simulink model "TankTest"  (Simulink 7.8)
settings: Solver=ode45  StartTime=0.0  StopTime=SimulationPeriod  RelTol=1e-7
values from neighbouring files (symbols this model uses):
  Ar1 = 1*2    (= 2)    [runSim.m]
  Ar2 = 0.6666667*2    (= 1.3333334)    [runSim.m]
  BT = 250-10*abs(8-i)    [runSim.m]
  g = 9.8    [runSim.m]
  h_add = 0.2    [runSim.m]
  k1 = 4.88e-4    (= 0.000488)    [runSim.m]
  k2 = 3.177e-4    (= 0.0003177)    [runSim.m]
  levelR1 = 1    [runSim.m]
  levelR2 = 0.75    [runSim.m]
  openloop = false    [runSim.m]
  qh0 = 0.01    [runSim.m]
  rho = 800    [runSim.m]
  Ttarget = 200    [runSim.m]
  UA0 = 100    [runSim.m]
undefined symbols (not defined in the file or in its folder): cp

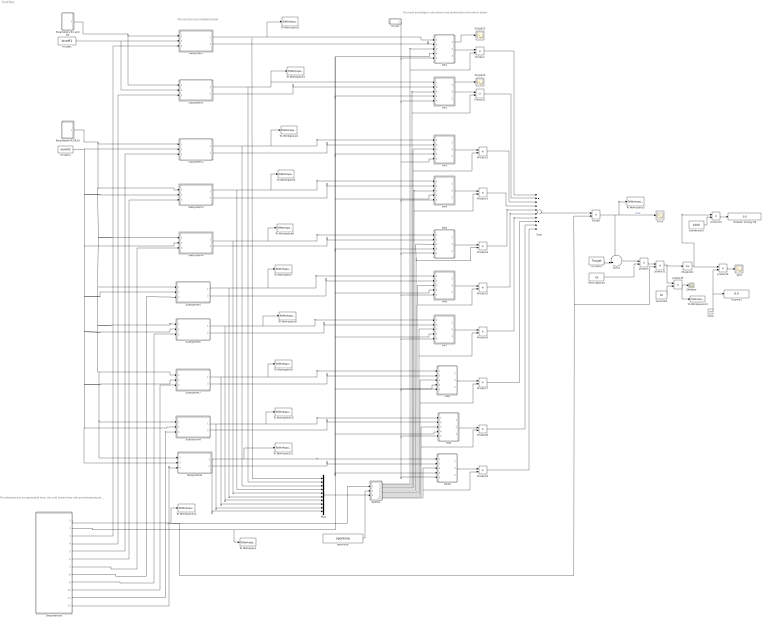
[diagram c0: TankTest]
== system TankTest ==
  note: The disturbances are generated here: the cold stream flow rate and temperatuere and the trigger times for the hot streams
  note: The reactore are modelled below.
  note: The heat exchangers calculations are performed in the blocks below
  Clock : Clock
  Display1 : Display
  Disturbances : Subsystem
  Divide : Product  Inputs=*/
  HX par : Subsystem
  HX1 : MATLAB Function  TreatAsAtomicUnit=on
  HX10 : MATLAB Function  TreatAsAtomicUnit=on
  HX2 : MATLAB Function  TreatAsAtomicUnit=on
  HX3 : MATLAB Function  TreatAsAtomicUnit=on
  HX4 : MATLAB Function  TreatAsAtomicUnit=on
  HX5 : MATLAB Function  TreatAsAtomicUnit=on
  HX6 : MATLAB Function  TreatAsAtomicUnit=on
  HX7 : MATLAB Function  TreatAsAtomicUnit=on
  HX8 : MATLAB Function  TreatAsAtomicUnit=on
  HX9 : MATLAB Function  TreatAsAtomicUnit=on
  Heaater energy MJ : Display
  Integrator : Integrator
  Mux : Mux  Inputs=10
  Parameters R1 and R2 : Subsystem
  Parameters R2/R10 : Subsystem
  Product{,1..9} (10 alike) : Product
  Qheater : Scope
  Qint : Scope
  Scope22 : Scope
  Scope23 : Scope
  Splitter : Subsystem
  Subsystem : Subsystem
  Subsystem1 : Subsystem
  Subsystem2 : Subsystem
  Subsystem3 : Subsystem
  Subsystem4 : Subsystem
  Subsystem5 : Subsystem
  Subsystem6 : Subsystem
  Subsystem7 : Subsystem
  Subsystem8 : Subsystem
  Subsystem9 : Subsystem
  Sum : Sum  Inputs=++++++++++
  Sum1 : Sum  Inputs=-+|
  Tmix : Scope
  To Workspace : ToWorkspace  VariableName=T0  SampleTime=-1  SaveFormat=Structure With Time
  To Workspace1 : ToWorkspace  VariableName=flowR1  SampleTime=-1  SaveFormat=Structure With Time
  To Workspace10 : ToWorkspace  VariableName=flowR9  SampleTime=-1  SaveFormat=Structure With Time
  To Workspace11 : ToWorkspace  VariableName=flowR10  SampleTime=-1  SaveFormat=Structure With Time
  To Workspace12 : ToWorkspace  VariableName=q0flow  SampleTime=-1  SaveFormat=Structure With Time
  To Workspace13 : ToWorkspace  VariableName=Qheater  SampleTime=-1  SaveFormat=Structure With Time
  To Workspace2 : ToWorkspace  VariableName=Tmix  SampleTime=-1  SaveFormat=Structure With Time
  To Workspace3 : ToWorkspace  VariableName=flowR2  SampleTime=-1  SaveFormat=Structure With Time
  To Workspace4 : ToWorkspace  VariableName=flowR3  SampleTime=-1  SaveFormat=Structure With Time
  To Workspace5 : ToWorkspace  VariableName=flowR4  SampleTime=-1  SaveFormat=Structure With Time
  To Workspace6 : ToWorkspace  VariableName=flowR5  SampleTime=-1  SaveFormat=Structure With Time
  To Workspace7 : ToWorkspace  VariableName=flowR6  SampleTime=-1  SaveFormat=Structure With Time
  To Workspace8 : ToWorkspace  VariableName=flowR7  SampleTime=-1  SaveFormat=Structure With Time
  To Workspace9 : ToWorkspace  VariableName=flowR8  SampleTime=-1  SaveFormat=Structure With Time
  converssion : Constant  Value=1000
  h1start : Constant  Value=levelR1
  h1start1 : Constant  Value=levelR2
  h1start2 : Constant  Value=Ttarget
  heat capacity : Constant  Value=cp
  openloop : Constant  Value=openloop
  product : Product  Inputs=**
  product1 : Product  Inputs=**
  product2 : Product  Inputs=*/
  product3 : Product  Inputs=*/
  product4 : Product  Inputs=*/
  seconds1 : Constant  Value=60
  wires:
  h1start/1 -> Subsystem/2(hstart), Subsystem1/2(hstart)
  Parameters R1 and R2/1(par 1) -> Subsystem/1(par), Subsystem1/1(par)
  h1start1/1 -> Subsystem8/2(hstart), Subsystem9/2(hstart), Subsystem7/2(hstart), Subsystem6/2(hstart), Subsystem5/2(hstart), Subsystem4/2(hstart), Subsystem3/2(hstart), Subsystem2/2(hstart)
  Parameters R2/R10/1(par 2) -> Subsystem8/1(par), Subsystem9/1(par), Subsystem7/1(par), Subsystem6/1(par), Subsystem5/1(par), Subsystem4/1(par), Subsystem3/1(par), Subsystem2/1(par)
  Disturbances/2(T0) -> To Workspace/1, HX2/4(Tcin), HX10/4(Tcin), HX9/4(Tcin), HX8/4(Tcin), HX7/4(Tcin), HX6/4(Tcin), HX5/4(Tcin), HX4/4(Tcin), HX3/4(Tcin), HX1/4(Tcin)
  Subsystem/2(Temperature) -> HX1/2(Thin)
  Subsystem/1(qh) -> Mux/1, HX1/1(qh), To Workspace1/1
  Subsystem1/1(qh) -> HX2/1(qh), To Workspace3/1, Mux/2
  Subsystem1/2(Temperature) -> HX2/2(Thin)
  Subsystem2/1(qh) -> HX3/1(qh), To Workspace4/1, Mux/3
  Subsystem2/2(Temperature) -> HX3/2(Thin)
  Subsystem3/1(qh) -> HX4/1(qh), To Workspace5/1, Mux/4
  Subsystem3/2(Temperature) -> HX4/2(Thin)
  Subsystem4/1(qh) -> HX5/1(qh), To Workspace6/1, Mux/5
  Subsystem4/2(Temperature) -> HX5/2(Thin)
  Subsystem5/1(qh) -> HX6/1(qh), To Workspace7/1, Mux/6
  Subsystem5/2(Temperature) -> HX6/2(Thin)
  Subsystem6/1(qh) -> HX7/1(qh), To Workspace8/1, Mux/7
  Subsystem6/2(Temperature) -> HX7/2(Thin)
  Subsystem7/1(qh) -> Mux/8, HX8/1(qh), To Workspace9/1
  Subsystem7/2(Temperature) -> HX8/2(Thin)
  Subsystem8/1(qh) -> Mux/9, HX9/1(qh), To Workspace10/1
  Subsystem8/2(Temperature) -> HX9/2(Thin)
  Subsystem9/1(qh) -> HX10/1(qh), To Workspace11/1, Mux/10
  Subsystem9/2(Temperature) -> HX10/2(Thin)
  HX par/1(par 1) -> HX10/5(par), HX9/5(par), HX8/5(par), HX7/5(par), HX6/5(par), HX5/5(par), HX4/5(par), HX3/5(par), HX2/5(par), HX1/5(par)
  Splitter/10(Out10) -> HX10/3(qc), Product9/2
  Splitter/9(Out9) -> HX9/3(qc), Product8/2
  Splitter/8(Out8) -> HX8/3(qc), Product7/2
  Splitter/7(Out7) -> HX7/3(qc), Product6/2
  Splitter/6(Out6) -> HX6/3(qc), Product5/2
  Splitter/5(Out5) -> HX5/3(qc), Product4/2
  Splitter/4(Out4) -> HX4/3(qc), Product3/2
  Splitter/3(Out3) -> HX3/3(qc), Product2/2
  Splitter/2(Out2) -> HX2/3(qc), Product1/2
  Splitter/1(Out1) -> HX1/3(qc), Product/2
  Disturbances/1(q0) -> Splitter/1(q0), Divide/2, product1/2, To Workspace12/1
  HX1/2(Tcout) -> Product/1
  HX2/2(Tcout) -> Product1/1
  HX4/2(Tcout) -> Product3/1
  HX5/2(Tcout) -> Product4/1
  HX6/2(Tcout) -> Product5/1
  HX7/2(Tcout) -> Product6/1
  HX8/2(Tcout) -> Product7/1
  HX9/2(Tcout) -> Product8/1
  HX10/2(Tcout) -> Product9/1
  Product/1 -> Sum/1
  Product1/1 -> Sum/2
  Product2/1 -> Sum/3
  Product3/1 -> Sum/4
  Product4/1 -> Sum/5
  Product5/1 -> Sum/6
  Product6/1 -> Sum/7
  Product7/1 -> Sum/8
  Product8/1 -> Sum/9
  Product9/1 -> Sum/10
  Sum/1 -> Divide/1
  Divide/1 -> Sum1/1, Tmix/1, To Workspace2/1  "Tmix"
  h1start2/1 -> Sum1/2
  Sum1/1 -> product/1
  heat capacity/1 -> product/2
  product/1 -> product1/1
  product1/1 -> Integrator/1, product4/1
  Integrator/1 -> product2/1, product3/1
  Disturbances/3(Trigger Batch 1) -> Subsystem/3(reset)
  Disturbances/4(Trigger Batch 2) -> Subsystem1/3(reset)
  Disturbances/5(Trigger Batch 3) -> Subsystem2/3(reset)
  Disturbances/6(Trigger Batch 4) -> Subsystem3/3(reset)
  Disturbances/7(Trigger Batch 5) -> Subsystem4/3(reset)
  Disturbances/8(Trigger Batch 6) -> Subsystem5/3(reset)
  Disturbances/9(Trigger Batch 7) -> Subsystem6/3(reset)
  Disturbances/11(Trigger Batch 9) -> Subsystem8/3(reset)
  Disturbances/12(Trigger Batch 10) -> Subsystem9/3(reset)
  HX3/2(Tcout) -> Product2/1
  Disturbances/10(Trigger Batch 8) -> Subsystem7/3(reset)
  Clock/1 -> product2/2, Display1/1
  product2/1 -> Qint/1
  Mux/1 -> Splitter/2(qh)
  converssion/1 -> product3/2
  product3/1 -> Heaater energy MJ/1
  seconds1/1 -> product4/2
  product4/1 -> Qheater/1, To Workspace13/1
  HX1/1(Thout) -> Scope22/1
  HX2/1(Thout) -> Scope23/1
  openloop/1 -> Splitter/3(control mode Openloop/ClosedLoop)

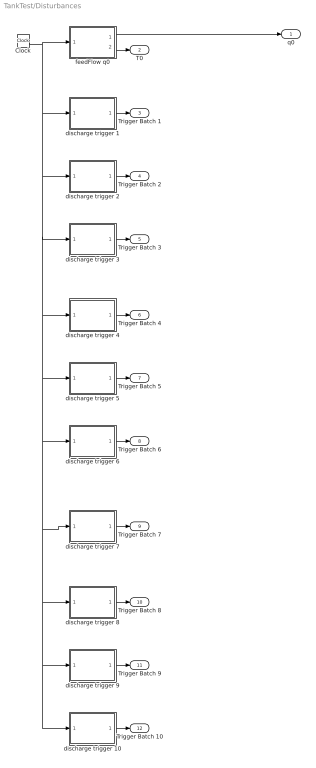
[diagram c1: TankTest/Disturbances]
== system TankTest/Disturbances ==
  Clock : Clock
  discharge trigger 1 : MATLAB Function  TreatAsAtomicUnit=on
  discharge trigger 10 : MATLAB Function  TreatAsAtomicUnit=on
  discharge trigger 2 : MATLAB Function  TreatAsAtomicUnit=on
  discharge trigger 3 : MATLAB Function  TreatAsAtomicUnit=on
  discharge trigger 4 : MATLAB Function  TreatAsAtomicUnit=on
  discharge trigger 5 : MATLAB Function  TreatAsAtomicUnit=on
  discharge trigger 6 : MATLAB Function  TreatAsAtomicUnit=on
  discharge trigger 7 : MATLAB Function  TreatAsAtomicUnit=on
  discharge trigger 8 : MATLAB Function  TreatAsAtomicUnit=on
  discharge trigger 9 : MATLAB Function  TreatAsAtomicUnit=on
  feedFlow q0 : MATLAB Function  TreatAsAtomicUnit=on
  q0 : Outport
  T0 : Outport  Port=2
  Trigger Batch 1 : Outport  Port=3
  Trigger Batch 2 : Outport  Port=4
  Trigger Batch 3 : Outport  Port=5
  Trigger Batch 4 : Outport  Port=6
  Trigger Batch 5 : Outport  Port=7
  Trigger Batch 6 : Outport  Port=8
  Trigger Batch 7 : Outport  Port=9
  Trigger Batch 8 : Outport  Port=10
  Trigger Batch 9 : Outport  Port=11
  Trigger Batch 10 : Outport  Port=12
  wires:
  Clock/1 -> feedFlow q0/1(time), discharge trigger 1/1(time), discharge trigger 2/1(time), discharge trigger 10/1(time), discharge trigger 9/1(time), discharge trigger 8/1(time), discharge trigger 7/1(time), discharge trigger 6/1(time), discharge trigger 5/1(time), discharge trigger 4/1(time), discharge trigger 3/1(time)
  feedFlow q0/1(q0) -> q0/1
  feedFlow q0/2(T0) -> T0/1
  discharge trigger 1/1(tr) -> Trigger Batch 1/1
  discharge trigger 2/1(tr) -> Trigger Batch 2/1
  discharge trigger 3/1(tr) -> Trigger Batch 3/1
  discharge trigger 4/1(tr) -> Trigger Batch 4/1
  discharge trigger 5/1(tr) -> Trigger Batch 5/1
  discharge trigger 6/1(tr) -> Trigger Batch 6/1
  discharge trigger 7/1(tr) -> Trigger Batch 7/1
  discharge trigger 8/1(tr) -> Trigger Batch 8/1
  discharge trigger 9/1(tr) -> Trigger Batch 9/1
  discharge trigger 10/1(tr) -> Trigger Batch 10/1

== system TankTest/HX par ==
  A2 : Constant  Value=cp
  Mux : Mux  Inputs=3
  Valve : Constant  Value=qh0
  rho2 : Constant  Value=UA0
  par 1 : Outport
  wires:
  Mux/1 -> par 1/1  "par"
  rho2/1 -> Mux/3
  A2/1 -> Mux/2
  Valve/1 -> Mux/1

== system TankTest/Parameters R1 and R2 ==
  Ar1 : Constant  Value=Ar1
  Mux : Mux  Inputs=5
  Valve : Constant  Value=k1
  g : Constant  Value=g
  h_add : Constant  Value=h_add
  rho : Constant  Value=rho
  par 1 : Outport
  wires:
  Valve/1 -> Mux/1
  Ar1/1 -> Mux/2
  rho/1 -> Mux/3
  h_add/1 -> Mux/4
  g/1 -> Mux/5
  Mux/1 -> par 1/1  "par"

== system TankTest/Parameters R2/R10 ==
  Ar2 : Constant  Value=Ar2
  Mux : Mux  Inputs=5
  Valve : Constant  Value=k2
  g : Constant  Value=g
  h_add : Constant  Value=h_add
  rho : Constant  Value=rho
  par 2 : Outport
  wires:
  Mux/1 -> par 2/1  "par"
  g/1 -> Mux/5
  h_add/1 -> Mux/4
  rho/1 -> Mux/3
  Ar2/1 -> Mux/2
  Valve/1 -> Mux/1

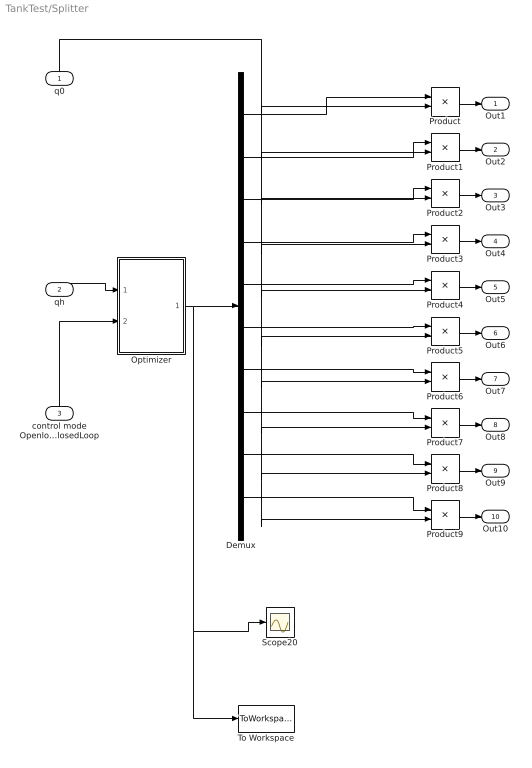
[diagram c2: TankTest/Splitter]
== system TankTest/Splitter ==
  q0 : Inport
  qh : Inport  Port=2
  control mode Openloop/ClosedLoop : Inport  Port=3
  Demux : Demux  Outputs=10
  Optimizer : MATLAB Function  TreatAsAtomicUnit=on
  Product{,1..9} (10 alike) : Product
  Scope20 : Scope
  To Workspace : ToWorkspace  VariableName=fractionfi  SampleTime=-1  SaveFormat=Structure With Time
  Out1 : Outport
  Out2 : Outport  Port=2
  Out3 : Outport  Port=3
  Out4 : Outport  Port=4
  Out5 : Outport  Port=5
  Out6 : Outport  Port=6
  Out7 : Outport  Port=7
  Out8 : Outport  Port=8
  Out9 : Outport  Port=9
  Out10 : Outport  Port=10
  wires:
  q0/1 -> Product/2, Product1/2, Product2/2, Product3/2, Product4/2, Product5/2, Product6/2, Product8/2, Product9/2, Product7/2
  Product/1 -> Out1/1
  Product1/1 -> Out2/1
  Product2/1 -> Out3/1
  Product3/1 -> Out4/1
  Product4/1 -> Out5/1
  Product5/1 -> Out6/1
  Product6/1 -> Out7/1
  Product7/1 -> Out8/1
  Product8/1 -> Out9/1
  Product9/1 -> Out10/1
  qh/1 -> Optimizer/1(qh)
  Optimizer/1(f) -> Demux/1, To Workspace/1, Scope20/1
  Demux/1 -> Product/1
  Demux/2 -> Product1/1
  Demux/3 -> Product2/1
  Demux/4 -> Product3/1
  Demux/5 -> Product4/1
  Demux/6 -> Product5/1
  Demux/7 -> Product6/1
  Demux/8 -> Product7/1
  Demux/9 -> Product8/1
  Demux/10 -> Product9/1
  control mode Openloop/ClosedLoop/1 -> Optimizer/2(openloop)

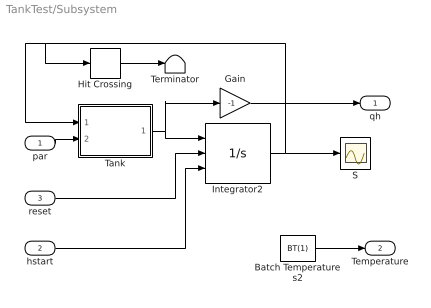
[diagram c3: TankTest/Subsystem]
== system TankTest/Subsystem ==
  par : Inport
  hstart : Inport  Port=2
  reset : Inport  Port=3
  Batch Temperatures2 : Constant  Value=BT(1)
  Gain : Gain  Gain=-1
  Hit Crossing : HitCross  HitCrossingDirection=falling
  Integrator2 : Integrator  ExternalReset=rising  InitialConditionSource=external
  S : Scope
  Tank : MATLAB Function  TreatAsAtomicUnit=on
  Terminator : Terminator
  qh : Outport
  Temperature : Outport  Port=2
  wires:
  Tank/1(f) -> Integrator2/1, Gain/1
  Integrator2/1 -> Tank/1(h), Hit Crossing/1, S/1
  par/1 -> Tank/2(par)
  reset/1 -> Integrator2/2
  hstart/1 -> Integrator2/3
  Gain/1 -> qh/1
  Hit Crossing/1 -> Terminator/1
  Batch Temperatures2/1 -> Temperature/1

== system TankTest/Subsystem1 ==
  par : Inport
  hstart : Inport  Port=2
  reset : Inport  Port=3
  Batch Temperatures2 : Constant  Value=BT(2)
  Gain : Gain  Gain=-1
  Hit Crossing : HitCross  HitCrossingDirection=falling
  Integrator2 : Integrator  ExternalReset=rising  InitialConditionSource=external
  Scope1 : Scope
  Tank : MATLAB Function  TreatAsAtomicUnit=on
  Terminator : Terminator
  qh : Outport
  Temperature : Outport  Port=2
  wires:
  Hit Crossing/1 -> Terminator/1
  Gain/1 -> qh/1
  hstart/1 -> Integrator2/3
  reset/1 -> Integrator2/2
  par/1 -> Tank/2(par)
  Integrator2/1 -> Hit Crossing/1, Tank/1(h), Scope1/1
  Tank/1(f) -> Gain/1, Integrator2/1
  Batch Temperatures2/1 -> Temperature/1

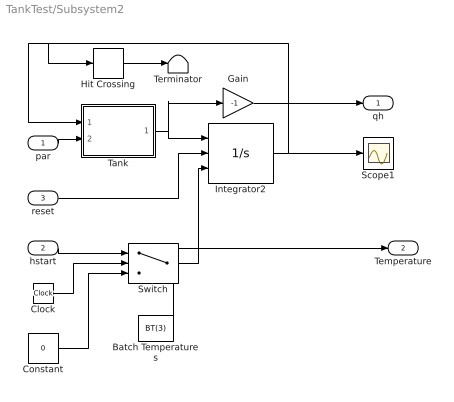
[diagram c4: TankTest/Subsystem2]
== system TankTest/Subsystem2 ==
  par : Inport
  hstart : Inport  Port=2
  reset : Inport  Port=3
  Batch Temperatures : Constant  Value=BT(3)
  Clock : Clock
  Constant : Constant  Value=0
  Gain : Gain  Gain=-1
  Hit Crossing : HitCross  HitCrossingDirection=falling
  Integrator2 : Integrator  ExternalReset=rising  InitialConditionSource=external
  Scope1 : Scope
  Switch : Switch  Threshold=2
  Tank : MATLAB Function  TreatAsAtomicUnit=on
  Terminator : Terminator
  qh : Outport
  Temperature : Outport  Port=2
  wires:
  Tank/1(f) -> Integrator2/1, Gain/1
  Integrator2/1 -> Tank/1(h), Hit Crossing/1, Scope1/1
  par/1 -> Tank/2(par)
  reset/1 -> Integrator2/2
  hstart/1 -> Switch/1
  Gain/1 -> qh/1
  Hit Crossing/1 -> Terminator/1
  Batch Temperatures/1 -> Temperature/1
  Clock/1 -> Switch/2
  Constant/1 -> Switch/3
  Switch/1 -> Integrator2/3

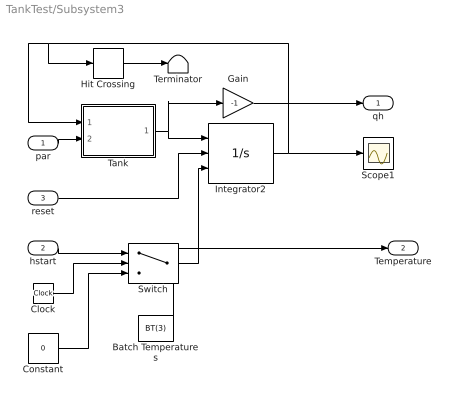
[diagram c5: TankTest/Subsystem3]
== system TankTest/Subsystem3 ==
  par : Inport
  hstart : Inport  Port=2
  reset : Inport  Port=3
  Batch Temperatures : Constant  Value=BT(3)
  Clock : Clock
  Constant : Constant  Value=0
  Gain : Gain  Gain=-1
  Hit Crossing : HitCross  HitCrossingDirection=falling
  Integrator2 : Integrator  ExternalReset=rising  InitialConditionSource=external
  Scope1 : Scope
  Switch : Switch  Threshold=2
  Tank : MATLAB Function  TreatAsAtomicUnit=on
  Terminator : Terminator
  qh : Outport
  Temperature : Outport  Port=2
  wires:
  Switch/1 -> Integrator2/3
  Constant/1 -> Switch/3
  Clock/1 -> Switch/2
  Batch Temperatures/1 -> Temperature/1
  Hit Crossing/1 -> Terminator/1
  Gain/1 -> qh/1
  hstart/1 -> Switch/1
  reset/1 -> Integrator2/2
  par/1 -> Tank/2(par)
  Integrator2/1 -> Scope1/1, Hit Crossing/1, Tank/1(h)
  Tank/1(f) -> Gain/1, Integrator2/1

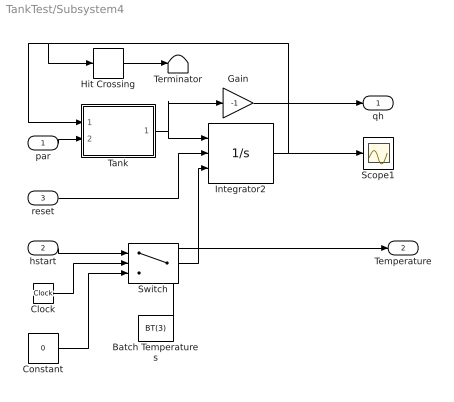
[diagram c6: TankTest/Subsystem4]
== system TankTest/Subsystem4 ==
  par : Inport
  hstart : Inport  Port=2
  reset : Inport  Port=3
  Batch Temperatures : Constant  Value=BT(3)
  Clock : Clock
  Constant : Constant  Value=0
  Gain : Gain  Gain=-1
  Hit Crossing : HitCross  HitCrossingDirection=falling
  Integrator2 : Integrator  ExternalReset=rising  InitialConditionSource=external
  Scope1 : Scope
  Switch : Switch  Threshold=2
  Tank : MATLAB Function  TreatAsAtomicUnit=on
  Terminator : Terminator
  qh : Outport
  Temperature : Outport  Port=2
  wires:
  Tank/1(f) -> Integrator2/1, Gain/1
  Integrator2/1 -> Tank/1(h), Hit Crossing/1, Scope1/1
  par/1 -> Tank/2(par)
  reset/1 -> Integrator2/2
  hstart/1 -> Switch/1
  Gain/1 -> qh/1
  Hit Crossing/1 -> Terminator/1
  Batch Temperatures/1 -> Temperature/1
  Clock/1 -> Switch/2
  Constant/1 -> Switch/3
  Switch/1 -> Integrator2/3

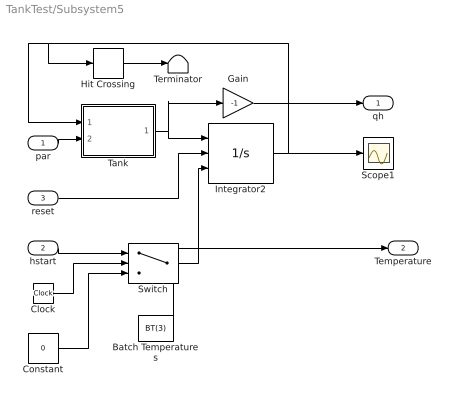
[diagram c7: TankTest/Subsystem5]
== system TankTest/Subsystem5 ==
  par : Inport
  hstart : Inport  Port=2
  reset : Inport  Port=3
  Batch Temperatures : Constant  Value=BT(3)
  Clock : Clock
  Constant : Constant  Value=0
  Gain : Gain  Gain=-1
  Hit Crossing : HitCross  HitCrossingDirection=falling
  Integrator2 : Integrator  ExternalReset=rising  InitialConditionSource=external
  Scope1 : Scope
  Switch : Switch  Threshold=2
  Tank : MATLAB Function  TreatAsAtomicUnit=on
  Terminator : Terminator
  qh : Outport
  Temperature : Outport  Port=2
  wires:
  Switch/1 -> Integrator2/3
  Constant/1 -> Switch/3
  Clock/1 -> Switch/2
  Batch Temperatures/1 -> Temperature/1
  Hit Crossing/1 -> Terminator/1
  Gain/1 -> qh/1
  hstart/1 -> Switch/1
  reset/1 -> Integrator2/2
  par/1 -> Tank/2(par)
  Integrator2/1 -> Scope1/1, Hit Crossing/1, Tank/1(h)
  Tank/1(f) -> Gain/1, Integrator2/1

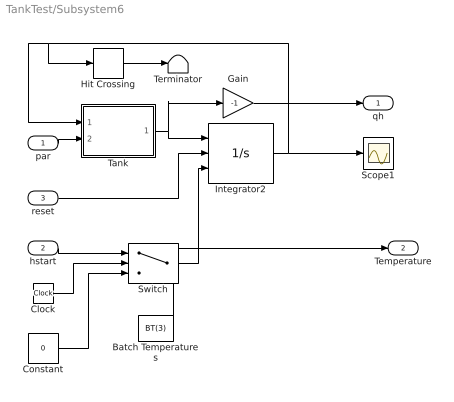
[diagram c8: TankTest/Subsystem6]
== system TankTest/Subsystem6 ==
  par : Inport
  hstart : Inport  Port=2
  reset : Inport  Port=3
  Batch Temperatures : Constant  Value=BT(3)
  Clock : Clock
  Constant : Constant  Value=0
  Gain : Gain  Gain=-1
  Hit Crossing : HitCross  HitCrossingDirection=falling
  Integrator2 : Integrator  ExternalReset=rising  InitialConditionSource=external
  Scope1 : Scope
  Switch : Switch  Threshold=2
  Tank : MATLAB Function  TreatAsAtomicUnit=on
  Terminator : Terminator
  qh : Outport
  Temperature : Outport  Port=2
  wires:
  Tank/1(f) -> Integrator2/1, Gain/1
  Integrator2/1 -> Tank/1(h), Hit Crossing/1, Scope1/1
  par/1 -> Tank/2(par)
  reset/1 -> Integrator2/2
  hstart/1 -> Switch/1
  Gain/1 -> qh/1
  Hit Crossing/1 -> Terminator/1
  Batch Temperatures/1 -> Temperature/1
  Clock/1 -> Switch/2
  Constant/1 -> Switch/3
  Switch/1 -> Integrator2/3

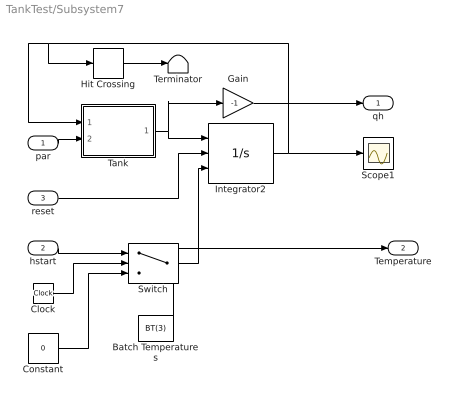
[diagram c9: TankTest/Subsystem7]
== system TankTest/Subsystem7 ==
  par : Inport
  hstart : Inport  Port=2
  reset : Inport  Port=3
  Batch Temperatures : Constant  Value=BT(3)
  Clock : Clock
  Constant : Constant  Value=0
  Gain : Gain  Gain=-1
  Hit Crossing : HitCross  HitCrossingDirection=falling
  Integrator2 : Integrator  ExternalReset=rising  InitialConditionSource=external
  Scope1 : Scope
  Switch : Switch  Threshold=2
  Tank : MATLAB Function  TreatAsAtomicUnit=on
  Terminator : Terminator
  qh : Outport
  Temperature : Outport  Port=2
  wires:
  Switch/1 -> Integrator2/3
  Constant/1 -> Switch/3
  Clock/1 -> Switch/2
  Batch Temperatures/1 -> Temperature/1
  Hit Crossing/1 -> Terminator/1
  Gain/1 -> qh/1
  hstart/1 -> Switch/1
  reset/1 -> Integrator2/2
  par/1 -> Tank/2(par)
  Integrator2/1 -> Scope1/1, Hit Crossing/1, Tank/1(h)
  Tank/1(f) -> Gain/1, Integrator2/1

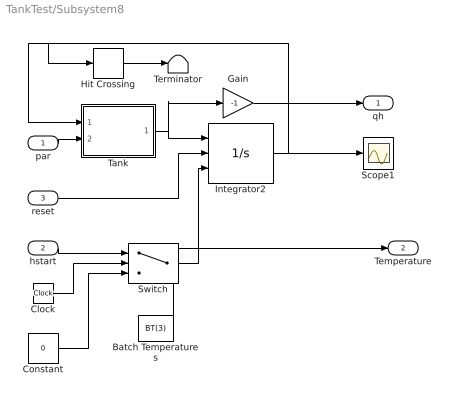
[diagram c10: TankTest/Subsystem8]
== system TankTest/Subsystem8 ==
  par : Inport
  hstart : Inport  Port=2
  reset : Inport  Port=3
  Batch Temperatures : Constant  Value=BT(3)
  Clock : Clock
  Constant : Constant  Value=0
  Gain : Gain  Gain=-1
  Hit Crossing : HitCross  HitCrossingDirection=falling
  Integrator2 : Integrator  ExternalReset=rising  InitialConditionSource=external
  Scope1 : Scope
  Switch : Switch  Threshold=2
  Tank : MATLAB Function  TreatAsAtomicUnit=on
  Terminator : Terminator
  qh : Outport
  Temperature : Outport  Port=2
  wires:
  Tank/1(f) -> Integrator2/1, Gain/1
  Integrator2/1 -> Tank/1(h), Hit Crossing/1, Scope1/1
  par/1 -> Tank/2(par)
  reset/1 -> Integrator2/2
  hstart/1 -> Switch/1
  Gain/1 -> qh/1
  Hit Crossing/1 -> Terminator/1
  Batch Temperatures/1 -> Temperature/1
  Clock/1 -> Switch/2
  Constant/1 -> Switch/3
  Switch/1 -> Integrator2/3

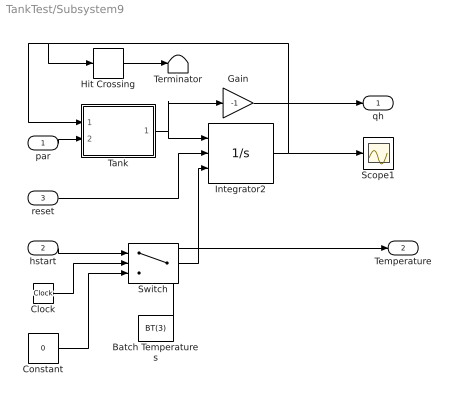
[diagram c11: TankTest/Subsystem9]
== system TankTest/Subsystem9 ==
  par : Inport
  hstart : Inport  Port=2
  reset : Inport  Port=3
  Batch Temperatures : Constant  Value=BT(3)
  Clock : Clock
  Constant : Constant  Value=0
  Gain : Gain  Gain=-1
  Hit Crossing : HitCross  HitCrossingDirection=falling
  Integrator2 : Integrator  ExternalReset=rising  InitialConditionSource=external
  Scope1 : Scope
  Switch : Switch  Threshold=2
  Tank : MATLAB Function  TreatAsAtomicUnit=on
  Terminator : Terminator
  qh : Outport
  Temperature : Outport  Port=2
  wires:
  Switch/1 -> Integrator2/3
  Constant/1 -> Switch/3
  Clock/1 -> Switch/2
  Batch Temperatures/1 -> Temperature/1
  Hit Crossing/1 -> Terminator/1
  Gain/1 -> qh/1
  hstart/1 -> Switch/1
  reset/1 -> Integrator2/2
  par/1 -> Tank/2(par)
  Integrator2/1 -> Scope1/1, Hit Crossing/1, Tank/1(h)
  Tank/1(f) -> Gain/1, Integrator2/1

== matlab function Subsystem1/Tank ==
function f = fcn(h,par)

% The right hand side of the differential equation for the reactor volume
k=par(1);
A=par(2);
rho = par(3);
h_add = par(4);
g =par(5);

if h>=0
    f = -k/A*sqrt(abs(rho*g*(h+h_add)));
else
    f=0;
end

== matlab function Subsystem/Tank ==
function f = fcn(h,par)

% The right hand side of the differential equation for the reactor volume
k=par(1);
A=par(2);
rho = par(3);
h_add = par(4);
g =par(5);

if h>=0
    f = -k/A*sqrt(abs(rho*g*(h+h_add)));
else
    f=0;
end

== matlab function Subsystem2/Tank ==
function f = fcn(h,par)

% The right hand side of the differential equation for the reactor volume
k=par(1);
A=par(2);
rho = par(3);
h_add = par(4);
g =par(5);

if h>=0
    f = -k/A*sqrt(abs(rho*g*(h+h_add)));
else
    f=0;
end

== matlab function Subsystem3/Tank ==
function f = fcn(h,par)

% The right hand side of the differential equation for the reactor volume
k=par(1);
A=par(2);
rho = par(3);
h_add = par(4);
g =par(5);

if h>=0
    f = -k/A*sqrt(abs(rho*g*(h+h_add)));
else
    f=0;
end

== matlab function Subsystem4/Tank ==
function f = fcn(h,par)

% The right hand side of the differential equation for the reactor volume
k=par(1);
A=par(2);
rho = par(3);
h_add = par(4);
g =par(5);

if h>=0
    f = -k/A*sqrt(abs(rho*g*(h+h_add)));
else
    f=0;
end

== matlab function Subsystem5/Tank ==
function f = fcn(h,par)

% The right hand side of the differential equation for the reactor volume
k=par(1);
A=par(2);
rho = par(3);
h_add = par(4);
g =par(5);

if h>=0
    f = -k/A*sqrt(abs(rho*g*(h+h_add)));
else
    f=0;
end

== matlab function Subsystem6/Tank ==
function f = fcn(h,par)

% The right hand side of the differential equation for the reactor volume
k=par(1);
A=par(2);
rho = par(3);
h_add = par(4);
g =par(5);

if h>=0
    f = -k/A*sqrt(abs(rho*g*(h+h_add)));
else
    f=0;
end

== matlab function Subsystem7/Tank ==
function f = fcn(h,par)

% The right hand side of the differential equation for the reactor volume
k=par(1);
A=par(2);
rho = par(3);
h_add = par(4);
g =par(5);

if h>=0
    f = -k/A*sqrt(abs(rho*g*(h+h_add)));
else
    f=0;
end

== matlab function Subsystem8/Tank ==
function f = fcn(h,par)

% The right hand side of the differential equation for the reactor volume
k=par(1);
A=par(2);
rho = par(3);
h_add = par(4);
g =par(5);

if h>=0
    f = -k/A*sqrt(abs(rho*g*(h+h_add)));
else
    f=0;
end

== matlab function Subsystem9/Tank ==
function f = fcn(h,par)

% The right hand side of the differential equation for the reactor volume
k=par(1);
A=par(2);
rho = par(3);
h_add = par(4);
g =par(5);

if h>=0
    f = -k/A*sqrt(abs(rho*g*(h+h_add)));
else
    f=0;
end

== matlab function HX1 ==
function [Thout, Tcout,Q] = fcn(qh,Thin,qc,Tcin,par)
% function to calculate the output temperatures as functions of the input
% temperatures.
qh0 =par(1);
cp = par(2);
threshold = 0.000001  ; 
UA0=par(3);


if qh<=threshold || qc<=threshold; % no heat transfer
    Tcout = Tcin;
    Thout = Thin;
    %aa='zero flow';
    
else
   C =qc/qh;
   UA=UA0*(qh/qh0)^0.8;
   NTU = UA/(qc*cp);
   %if 0.9999<=C<=1.0001
   %    ec=NTU/(NTU+1);
   %    eh = ec;
   %else
       E = -NTU*(C-1);
       ec = (1-exp(E))/(C-exp(E));
       eh = C*ec;
   %end
   Thout = (1-eh)*Thin + eh*Tcin;
   Tcout = ec*Thin+(1-ec)*Tcin;
end
Q=qh*cp*(Thin-Thout);
end

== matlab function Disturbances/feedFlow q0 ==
function [q0,T0] = fcn(time)
%#Function to generate the sequence of flow disturbances
% Johannes Jaeschke


q0 = 0.1/2; %m3
delta_q = 0.05/2;

period1 = 1.8*60;
dpaux1 = period1/2;
n1 = time/dpaux1;
n1=floor(n1);

if mod(n1,2)==1
    q0 =q0+delta_q;
end

% The temperature disturbances for the cold stream
T0basic = 70;
delta_T = 10;
period2 = 4*60;
dpaux2= period2/4;

n2 = time/dpaux2;
n2 = floor(n2);

if mod(n2,4) == 1
    T0=T0basic+delta_T;
elseif mod(n2,4) == 2 
    T0 =T0basic;
elseif mod(n2,4) == 3 
    T0 =T0basic-delta_T;
else% mod(n2,4) == 0 
    T0 =T0basic;
end

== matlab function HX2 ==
function [Thout, Tcout,Q] = fcn(qh,Thin,qc,Tcin,par)
% function to calculate the output temperatures as functions of the input
% temperatures.
qh0 =par(1);
cp = par(2);
threshold = 0.000001  ; 
UA0=par(3);

if qh<=threshold || qc<=threshold; % no heat transfer
    Tcout = Tcin;
    Thout = Thin;
    
    
else
   C =qc/qh;
   UA=UA0*(qh/qh0)^0.8;
   NTU = UA/(qc*cp);
   %if 0.9999<=C<=1.0001
   %    ec=NTU/(NTU+1);
   %    eh = ec;
   %else
       E = -NTU*(C-1);
       ec = (1-exp(E))/(C-exp(E));
       eh = C*ec;
   %end
   Thout = (1-eh)*Thin + eh*Tcin;
   Tcout = ec*Thin+(1-ec)*Tcin;
end
Q=qh*cp*(Thin-Thout);
end

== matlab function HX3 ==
function [Thout, Tcout,Q] = fcn(qh,Thin,qc,Tcin,par)
% function to calculate the output temperatures as functions of the input
% temperatures.
qh0 =par(1);
cp = par(2);
threshold = 0.000001  ; 

UA0=par(3);
if qh<=threshold || qc<=threshold; % no heat transfer
    Tcout = Tcin;
    Thout = Thin;
 
    
else
   C =qc/qh;
   UA=UA0*(qh/qh0)^0.8;
   NTU = UA/(qc*cp);
   %if 0.9999<=C<=1.0001
   %    ec=NTU/(NTU+1);
   %    eh = ec;
   %else
       E = -NTU*(C-1);
       ec = (1-exp(E))/(C-exp(E));
       eh = C*ec;
   %end
   Thout = (1-eh)*Thin + eh*Tcin;
   Tcout = ec*Thin+(1-ec)*Tcin;
end
Q=qh*cp*(Thin-Thout);
%DTc = Tcout-Tcin;
end

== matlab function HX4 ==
function [Thout, Tcout,Q] = fcn(qh,Thin,qc,Tcin,par)
% function to calculate the output temperatures as functions of the input
% temperatures.
qh0 =par(1);
cp = par(2);
threshold = 0.000001  ; 

UA0=par(3);
if qh<=threshold || qc<=threshold; % no heat transfer
    Tcout = Tcin;
    Thout = Thin;

    
else
   C =qc/qh;
   UA=UA0*(qh/qh0)^0.8;
   NTU = UA/(qc*cp);
   %if 0.9999<=C<=1.0001
   %    ec=NTU/(NTU+1);
   %    eh = ec;
   %else
       E = -NTU*(C-1);
       ec = (1-exp(E))/(C-exp(E));
       eh = C*ec;
   %end
   Thout = (1-eh)*Thin + eh*Tcin;
   Tcout = ec*Thin+(1-ec)*Tcin;
end
Q=qh*cp*(Thin-Thout);
end

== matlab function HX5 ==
function [Thout, Tcout,Q] = fcn(qh,Thin,qc,Tcin,par)
% function to calculate the output temperatures as functions of the input
% temperatures.
qh0 =par(1);
cp = par(2);
threshold = 0.000001  ; 
UA0=par(3);

if qh<=threshold || qc<=threshold; % no heat transfer
    Tcout = Tcin;
    Thout = Thin;
    
else
   C =qc/qh;
   UA=UA0*(qh/qh0)^0.8;
   NTU = UA/(qc*cp);
   %if 0.9999<=C<=1.0001
   %    ec=NTU/(NTU+1);
   %    eh = ec;
   %else
       E = -NTU*(C-1);
       ec = (1-exp(E))/(C-exp(E));
       eh = C*ec;
   %end
   Thout = (1-eh)*Thin + eh*Tcin;
   Tcout = ec*Thin+(1-ec)*Tcin;
end
Q=qh*cp*(Thin-Thout);
end

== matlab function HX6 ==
function [Thout, Tcout,Q] = fcn(qh,Thin,qc,Tcin,par)
% function to calculate the output temperatures as functions of the input
% temperatures.
qh0 =par(1);
cp = par(2);
threshold = 0.000001  ; 

UA0=par(3);
if qh<=threshold || qc<=threshold; % no heat transfer
    Tcout = Tcin;
    Thout = Thin;

    
else
   C =qc/qh;
   UA=UA0*(qh/qh0)^0.8;
   NTU = UA/(qc*cp);
   %if 0.9999<=C<=1.0001
   %    ec=NTU/(NTU+1);
   %    eh = ec;
   %else
       E = -NTU*(C-1);
       ec = (1-exp(E))/(C-exp(E));
       eh = C*ec;
   %end
   Thout = (1-eh)*Thin + eh*Tcin;
   Tcout = ec*Thin+(1-ec)*Tcin;
end
Q=qh*cp*(Thin-Thout);
end

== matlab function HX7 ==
function [Thout, Tcout,Q] = fcn(qh,Thin,qc,Tcin,par)
% function to calculate the output temperatures as functions of the input
% temperatures.
qh0 =par(1);
cp = par(2);
threshold = 0.000001  ; 
UA0=par(3);


if qh<=threshold || qc<=threshold; % no heat transfer
    Tcout = Tcin;
    Thout = Thin;

    
else
   C =qc/qh;
   UA=UA0*(qh/qh0)^0.8;
   NTU = UA/(qc*cp);
   %if 0.9999<=C<=1.0001
   %    ec=NTU/(NTU+1);
   %    eh = ec;
   %else
       E = -NTU*(C-1);
       ec = (1-exp(E))/(C-exp(E));
       eh = C*ec;
   %end
   Thout = (1-eh)*Thin + eh*Tcin;
   Tcout = ec*Thin+(1-ec)*Tcin;
end
Q=qh*cp*(Thin-Thout);
end

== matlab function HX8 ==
function [Thout, Tcout,Q] = fcn(qh,Thin,qc,Tcin,par)
% function to calculate the output temperatures as functions of the input
% temperatures.
qh0 =par(1);
cp = par(2);
threshold = 0.000001  ; 

UA0=par(3);
if qh<=threshold || qc<=threshold; % no heat transfer
    Tcout = Tcin;
    Thout = Thin;
    
else
   C =qc/qh;
   UA=UA0*(qh/qh0)^0.8;
   NTU = UA/(qc*cp);
   %if 0.9999<=C<=1.0001
   %    ec=NTU/(NTU+1);
   %    eh = ec;
   %else
       E = -NTU*(C-1);
       ec = (1-exp(E))/(C-exp(E));
       eh = C*ec;
   %end
   Thout = (1-eh)*Thin + eh*Tcin;
   Tcout = ec*Thin+(1-ec)*Tcin;
end
Q=qh*cp*(Thin-Thout);
end

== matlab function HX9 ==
function [Thout, Tcout,Q] = fcn(qh,Thin,qc,Tcin,par)
% function to calculate the output temperatures as functions of the input
% temperatures.
qh0 =par(1);
cp = par(2);
threshold = 0.000001  ; 

UA0=par(3);
if qh<=threshold || qc<=threshold; % no heat transfer
    Tcout = Tcin;
    Thout = Thin;

    
else
   C =qc/qh;
   UA=UA0*(qh/qh0)^0.8;
   NTU = UA/(qc*cp);
   %if 0.9999<=C<=1.0001
   %    ec=NTU/(NTU+1);
   %    eh = ec;
   %else
       E = -NTU*(C-1);
       ec = (1-exp(E))/(C-exp(E));
       eh = C*ec;
   %end
   Thout = (1-eh)*Thin + eh*Tcin;
   Tcout = ec*Thin+(1-ec)*Tcin;
end
Q=qh*cp*(Thin-Thout);
end

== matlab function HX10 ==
function [Thout, Tcout,Q] = fcn(qh,Thin,qc,Tcin,par)
% function to calculate the output temperatures as functions of the input
% temperatures.
qh0 =par(1);
cp = par(2);
threshold = 0.000001  ; 
UA0=par(3);

if qh<=threshold || qc<=threshold; % no heat transfer
    Tcout = Tcin;
    Thout = Thin;

    
else
   C =qc/qh;
   UA=UA0*(qh/qh0)^0.8;
   NTU = UA/(qc*cp);
   %if 0.9999<=C<=1.0001
   %    ec=NTU/(NTU+1);
   %    eh = ec;
   %else
       E = -NTU*(C-1);
       ec = (1-exp(E))/(C-exp(E));
       eh = C*ec;
   %end
   Thout = (1-eh)*Thin + eh*Tcin;
   Tcout = ec*Thin+(1-ec)*Tcin;
end
Q=qh*cp*(Thin-Thout);
end

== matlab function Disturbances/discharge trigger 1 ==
function tr  = fcn(time)
%#Function to generate the sequence of flow disturbances
% Johannes Jaeschke
%%%%%%%%%%%%%%%%%%%%%%%%%%%%%%%%%%%%%%%%%%%%%%%%%%%%%%%%%%5
% Change here:
% Trigger signal for discharging reactor i
%Reactor 1
ts1 =0;             % start time
deltaTtr = 210;     % time between discharges
%%%%%%%%%%%%%%%%%%%%%%%%%%%%%%%%%%%%%%%%%%%%%%%%%%%%5

%%%%%%%%%%%%%%%%%%%%%%%%%%%%%%%%%%%%%%%%%%%%%%%%%%%%%%
% Do not change this
tr         = 0;     % default 
% Divide period in half, 
dTtrhalv = deltaTtr/2;
tshift = time -ts1;
% the first trigger
if time>=ts1
    tr =1;
end
if time >ts1 && tshift >= 0
    n = floor(tshift/dTtrhalv);
    if mod(n,2)==0
        tr=1;
    else
        tr=0;
    end %if
end %if

end % function

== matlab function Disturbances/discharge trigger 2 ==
function tr  = fcn(time)
%#Function to generate the sequence of flow disturbances
% Johannes Jaeschke
% Reactor 2
%%%%%%%%%%%%%%%%%%%%%%%%%%%%%%%%%%%%%%%%%%%%%%%%%%%%%%%%%%5
% Change here:
% Reactor 2
% Trigger signal for discharging reactor i
ts1 =0;             % start time
deltaTtr = 225;     % time between discharges
%%%%%%%%%%%%%%%%%%%%%%%%%%%%%%%%%%%%%%%%%%%%%%%%%%%%5

%%%%%%%%%%%%%%%%%%%%%%%%%%%%%%%%%%%%%%%%%%%%%%%%%%%%%%
% Do not change this
tr         = 0;     % default 
% Divide period in half, 
dTtrhalv = deltaTtr/2;
tshift = time -ts1;
% the first trigger
if time>=ts1
    tr =1;
end
if time >ts1 && tshift >= 0
    n = floor(tshift/dTtrhalv);
    if mod(n,2)==0
        tr=1;
    else
        tr=0;
    end %if
end %if

end % function

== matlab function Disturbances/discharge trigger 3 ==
function tr  = fcn(time)
%#Function to generate the sequence of flow disturbances
% Johannes Jaeschke
%%%%%%%%%%%%%%%%%%%%%%%%%%%%%%%%%%%%%%%%%%%%%%%%%%%%%%%%%%5
% Change here:
% Trigger signal for discharging reactor i
% Reactor 3
ts1 =60;             % start time (20i)
deltaTtr = 240;     % time between discharges
%%%%%%%%%%%%%%%%%%%%%%%%%%%%%%%%%%%%%%%%%%%%%%%%%%%%5

%%%%%%%%%%%%%%%%%%%%%%%%%%%%%%%%%%%%%%%%%%%%%%%%%%%%%%
% Do not change this
tr         = 0;     % default 
% Divide period in half, 
dTtrhalv = deltaTtr/2;
tshift = time -ts1;
% the first trigger
if time>=ts1
    tr =1;
end
if time >ts1 && tshift >= 0
    n = floor(tshift/dTtrhalv);
    if mod(n,2)==0
        tr=1;
    else
        tr=0;
    end %if
end %if

end % function

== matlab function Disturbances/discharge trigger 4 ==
function tr  = fcn(time)
%#Function to generate the sequence of flow disturbances
% Johannes Jaeschke
%%%%%%%%%%%%%%%%%%%%%%%%%%%%%%%%%%%%%%%%%%%%%%%%%%%%%%%%%%5
% Change here:
% Trigger signal for discharging reactor i
%Reactor 4
ts1 =80;             % start time
deltaTtr = 225;     % time between discharges
%%%%%%%%%%%%%%%%%%%%%%%%%%%%%%%%%%%%%%%%%%%%%%%%%%%%5

%%%%%%%%%%%%%%%%%%%%%%%%%%%%%%%%%%%%%%%%%%%%%%%%%%%%%%
% Do not change this
tr         = 0;     % default 
% Divide period in half, 
dTtrhalv = deltaTtr/2;
tshift = time -ts1;
% the first trigger
if time>=ts1
    tr =1;
end
if time >ts1 && tshift >= 0
    n = floor(tshift/dTtrhalv);
    if mod(n,2)==0
        tr=1;
    else
        tr=0;
    end %if
end %if

end % function

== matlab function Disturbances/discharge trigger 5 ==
function tr  = fcn(time)
%#Function to generate the sequence of flow disturbances
% Johannes Jaeschke
% Reactor 2
%%%%%%%%%%%%%%%%%%%%%%%%%%%%%%%%%%%%%%%%%%%%%%%%%%%%%%%%%%5
% Change here:
% Trigger signal for discharging reactor i
% Reactor 5
ts1 =100;             % start time
deltaTtr = 210;     % time between discharges
%%%%%%%%%%%%%%%%%%%%%%%%%%%%%%%%%%%%%%%%%%%%%%%%%%%%5

%%%%%%%%%%%%%%%%%%%%%%%%%%%%%%%%%%%%%%%%%%%%%%%%%%%%%%
% Do not change this
tr         = 0;     % default 
% Divide period in half, 
dTtrhalv = deltaTtr/2;
tshift = time -ts1;
% the first trigger
if time>=ts1
    tr =1;
end
if time >ts1 && tshift >= 0
    n = floor(tshift/dTtrhalv);
    if mod(n,2)==0
        tr=1;
    else
        tr=0;
    end %if
end %if

end % function

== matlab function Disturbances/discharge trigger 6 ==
function tr  = fcn(time)
%#Function to generate the sequence of flow disturbances
% Johannes Jaeschke
%%%%%%%%%%%%%%%%%%%%%%%%%%%%%%%%%%%%%%%%%%%%%%%%%%%%%%%%%%5
% Change here:
% Trigger signal for discharging reactor i
% Reactor 6
ts1 =120;             % start time
deltaTtr = 195;     % time between discharges
%%%%%%%%%%%%%%%%%%%%%%%%%%%%%%%%%%%%%%%%%%%%%%%%%%%%5

%%%%%%%%%%%%%%%%%%%%%%%%%%%%%%%%%%%%%%%%%%%%%%%%%%%%%%
% Do not change this
tr         = 0;     % default 
% Divide period in half, 
dTtrhalv = deltaTtr/2;
tshift = time -ts1;
% the first trigger
if time>=ts1
    tr =1;
end
if time >ts1 && tshift >= 0
    n = floor(tshift/dTtrhalv);
    if mod(n,2)==0
        tr=1;
    else
        tr=0;
    end %if
end %if

end % function

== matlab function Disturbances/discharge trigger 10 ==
function tr  = fcn(time)
%#Function to generate the sequence of flow disturbances
% Johannes Jaeschke
%%%%%%%%%%%%%%%%%%%%%%%%%%%%%%%%%%%%%%%%%%%%%%%%%%%%%%%%%%5
% Change here:
% Trigger signal for discharging reactor i
% Reactor 10
ts1 =200;             % start time
deltaTtr = 135;     % time between discharges
%%%%%%%%%%%%%%%%%%%%%%%%%%%%%%%%%%%%%%%%%%%%%%%%%%%%5

%%%%%%%%%%%%%%%%%%%%%%%%%%%%%%%%%%%%%%%%%%%%%%%%%%%%%%
% Do not change this
tr         = 0;     % default 
% Divide period in half, 
dTtrhalv = deltaTtr/2;
tshift = time -ts1;
% the first trigger
if time>=ts1
    tr =1;
end
if time >ts1 && tshift >= 0
    n = floor(tshift/dTtrhalv);
    if mod(n,2)==0
        tr=1;
    else
        tr=0;
    end %if
end %if

end % function

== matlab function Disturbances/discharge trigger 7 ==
function tr  = fcn(time)
%#Function to generate the sequence of flow disturbances
% Johannes Jaeschke
%%%%%%%%%%%%%%%%%%%%%%%%%%%%%%%%%%%%%%%%%%%%%%%%%%%%%%%%%%5
% Change here:
% Trigger signal for discharging reactor i
% Reactor 7
ts1 =140;             % start time
deltaTtr = 180;     % time between discharges
%%%%%%%%%%%%%%%%%%%%%%%%%%%%%%%%%%%%%%%%%%%%%%%%%%%%5

%%%%%%%%%%%%%%%%%%%%%%%%%%%%%%%%%%%%%%%%%%%%%%%%%%%%%%
% Do not change this
tr         = 0;     % default 
% Divide period in half, 
dTtrhalv = deltaTtr/2;
tshift = time -ts1;
% the first trigger
if time>=ts1
    tr =1;
end
if time >ts1 && tshift >= 0
    n = floor(tshift/dTtrhalv);
    if mod(n,2)==0
        tr=1;
    else
        tr=0;
    end %if
end %if

end % function

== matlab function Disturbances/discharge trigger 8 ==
function tr  = fcn(time)
%#Function to generate the sequence of flow disturbances
% Johannes Jaeschke
%%%%%%%%%%%%%%%%%%%%%%%%%%%%%%%%%%%%%%%%%%%%%%%%%%%%%%%%%%5
% Change here:
% Trigger signal for discharging reactor i
%Reactor 8
ts1 =160;             % start time
deltaTtr = 165;     % time between discharges
%%%%%%%%%%%%%%%%%%%%%%%%%%%%%%%%%%%%%%%%%%%%%%%%%%%%5

%%%%%%%%%%%%%%%%%%%%%%%%%%%%%%%%%%%%%%%%%%%%%%%%%%%%%%
% Do not change this
tr         = 0;     % default 
% Divide period in half, 
dTtrhalv = deltaTtr/2;
tshift = time -ts1;
% the first trigger
if time>=ts1
    tr =1;
end
if time >ts1 && tshift >= 0
    n = floor(tshift/dTtrhalv);
    if mod(n,2)==0
        tr=1;
    else
        tr=0;
    end %if
end %if

end % function

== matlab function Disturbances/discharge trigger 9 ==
function tr = fcn(time)

%#Function to generate the sequence of flow disturbances
% Johannes Jaeschke
% Reactor 2
%%%%%%%%%%%%%%%%%%%%%%%%%%%%%%%%%%%%%%%%%%%%%%%%%%%%%%%%%%5
% Change here:
% Trigger signal for discharging reactor i
% Reactor 9
ts1 =180;             % start time
deltaTtr = 150;     % time between discharges
%%%%%%%%%%%%%%%%%%%%%%%%%%%%%%%%%%%%%%%%%%%%%%%%%%%%5

%%%%%%%%%%%%%%%%%%%%%%%%%%%%%%%%%%%%%%%%%%%%%%%%%%%%%%
% Do not change this
tr         = 0;     % default 
% Divide period in half, 
dTtrhalv = deltaTtr/2;
tshift = time -ts1;
% the first trigger
if time>=ts1
    tr =1;
end
if time >ts1 && tshift >= 0
    n = floor(tshift/dTtrhalv);
    if mod(n,2)==0
        tr=1;
    else
        tr=0;
    end %if
end %if

end % function

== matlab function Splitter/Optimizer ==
function f  = fcn(qh,openloop)
% function to calculate the split fractions
f=zeros(10,1);  % initialize the fractions
idx = find(qh>= 0.01);
nopen = numel(idx);

if openloop==true
    f=ones(10,1)/10;
else % "Optimize"
    if nopen == 0
        f= ones(10,1)/10;
    else
        f(idx)=1/nopen;
    end
end
% set equal split ratios
%f= ones(10,1)/10;
